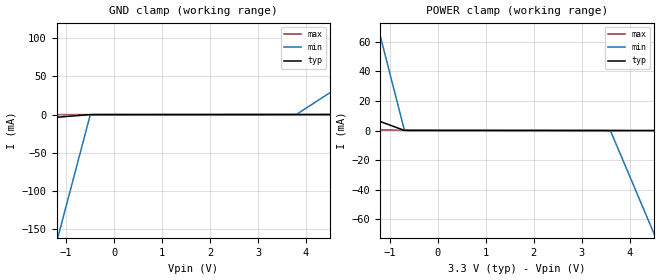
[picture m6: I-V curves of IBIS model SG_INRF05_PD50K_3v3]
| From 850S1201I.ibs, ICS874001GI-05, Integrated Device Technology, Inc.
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[Model] SG_INRF05_PD50K_3v3
Model_type   Input
Polarity   Non-Inverting
Vinl = 0.80V
Vinh = 2.2V
|   typ   min   max
C_comp   2pF   1.5pF   2.5pF
|   typ   min   max
[Voltage range]  3.3V   3.135V   3.465V
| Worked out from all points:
|   GND clamp passes 1 mA (typ) near -0.69 V on its own axis
|   POWER clamp passes 1 mA (typ) near -0.78 V on its own axis
[GND_clamp]
|Voltage   I(typ)   I(min)   I(max)
-3.3V     -14.17mA   -667.3mA   -213.1uA
-1.2V     -3.557mA   -167.5mA   -60.41uA
-1.1V     -3.052mA   -143.8mA   -53.14uA
-500mV    -20.42uA   -979.9uA   -9.515uA
-300mV    -5.971uA   -7.682uA   -5.679uA
3.8V      75.66uA    244.4uA    72.01uA
6.6V      145.4uA    114.2mA    125.2uA
[POWER_clamp]
|Voltage   I(typ)   I(min)   I(max)
-3.3V     31.08mA    329.4mA    2.044mA
-1.3V     7.253mA    76.48mA    532.9uA
-1.2V     6.062mA    63.84mA    457.3uA
-700mV    104.4uA    594.6uA    79.63uA
-500mV    75.66uA    75.93uA    75.14uA
3.6V      -5.971uA   -321.5uA   -2.555uA
4.5V      -25.75uA   -69.23mA   -19.59uA
4.6V      -27.95uA   -76.89mA   -21.48uA
6.6V      -71.92uA   -230mA     -59.34uA
